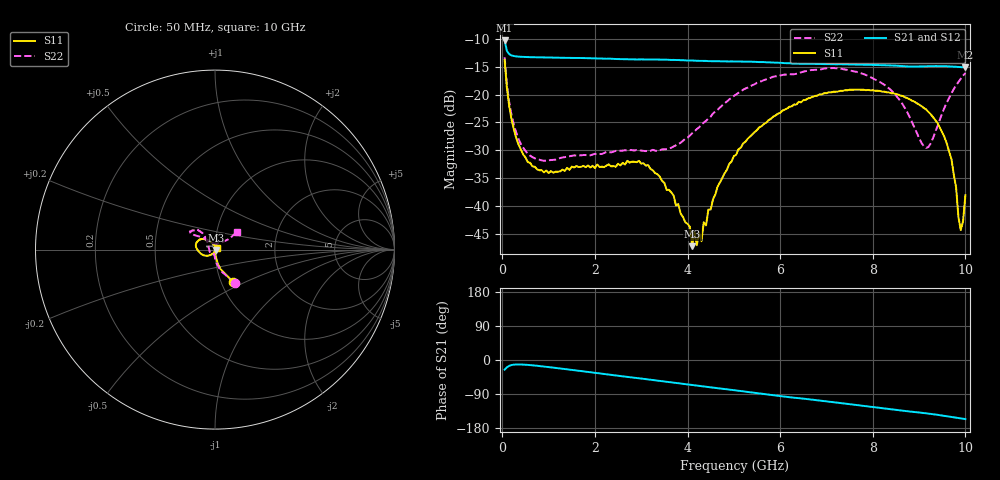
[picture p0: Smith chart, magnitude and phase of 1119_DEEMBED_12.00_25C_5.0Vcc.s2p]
!Hittite Microwave Corp.
!Digital Attenuator/PhaseShifter Rev 1.4.0
!Filename: C:\DATA\DATA\1119_DEEMBED_12.00_25C_5.0Vcc.s2p
!VNA ID: Agilent Technologies,N5224A,MY51441122,A.10.45.03
!Device type:
!2 Port Calibration.
!Temp(C): 25
!Lot Number:
!Serial Number:
!Operator:
!Misc:
!Attenuator:  12.000
# GHZ S DB R 50.0
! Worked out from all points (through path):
!   200 points, 50 MHz to 10 GHz, reference 50 ohm
!   highest |S21| = -10.29 dB at 50 MHz (marker M1); lowest = -15.1 dB at 10 GHz (marker M2)
!   group delay of S21, straight-line fit = 41.3 ps
!   lowest |S11| = -47.2 dB at 4.1 GHz (marker M3), VSWR 1.01, Z = 50.4 - j0.159 ohm
!   |S11| at or under -10 dB: start of sweep to end of sweep
!   |S22| runs from -31.9 to -13.3 dB; largest |S21 - S12| = 0.00055
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0.05  -13.76 -60.9  -10.29 -25.4  -10.28 -25.4  -13.30 -59.5
0.15  -22.09 -78.7  -12.75 -15.3  -12.75 -15.3  -21.42 -81.3
0.25  -26.25 -82.1  -13.09 -12.3  -13.10 -12.3  -25.43 -88.3
0.55  -32.12 -86.1  -13.27 -12.9  -13.27 -12.9  -30.57 -97.6
1.75  -32.79 -100.6  -13.45 -29.9  -13.45 -30.0  -30.85 -114.0
2.95  -31.90 -89.8  -13.69 -48.1  -13.69 -48.2  -30.01 -151.3
3.4  -34.72 -85.9  -13.72 -55.2  -13.73 -55.3  -29.98 -173.5
4.05  -43.72 -42.6  -13.88 -65.4  -13.89 -65.5  -27.37 150.6
4.1  -47.21 -21.2  -13.89 -66.3  -13.90 -66.3  -26.95 148.5
4.15  -44.64 -12.7  -13.91 -67.1  -13.92 -67.2  -26.60 145.9
4.2  -47.04 9.6  -13.94 -67.8  -13.95 -67.9  -26.19 143.6
4.25  -44.78 15.3  -13.95 -68.5  -13.96 -68.6  -25.90 142.0
4.3  -46.32 36.9  -13.96 -69.2  -13.98 -69.3  -25.37 140.2
4.35  -42.92 44.3  -13.96 -69.9  -13.97 -69.9  -25.03 138.2
4.65  -36.48 85.3  -14.01 -74.4  -14.03 -74.4  -22.73 130.9
5.05  -30.79 105.1  -14.07 -80.3  -14.08 -80.4  -19.97 127.1
6.7  -20.41 142.5  -14.49 -104.8  -14.50 -104.8  -15.58 139.9
8.35  -19.61 174.4  -14.77 -129.6  -14.77 -129.6  -18.89 139.8
9.15  -22.65 -156.0  -14.93 -140.7  -14.94 -140.7  -29.57 89.4
9.7  -31.62 -118.8  -14.96 -150.3  -14.97 -150.3  -19.76 37.4
9.9  -44.33 -42.0  -15.07 -154.1  -15.08 -154.1  -17.16 38.4
10  -38.06 38.1  -15.14 -155.9  -15.15 -155.9  -16.13 39.2
